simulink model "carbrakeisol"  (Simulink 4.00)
settings: Solver=ode15s  StartTime=0.0  StopTime=Te  RelTol=1e-3
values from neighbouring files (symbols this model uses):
  c1 = 500    [bspbesch.m]    (also in bspofen.m = 921; carbrake.m = 0.857; ffwfback.m = [1 0]; kennwrt.m = 1)
  c2 = 921    [bspbesch.m]    (also in bspofen.m = 465; carbrake.m = 33.822; kennwrt.m = 1; schlupfsoll.m = 33.822)
  c3 = 465    [bspbesch.m]    (also in carbrake.m = 0.347; schlupfsoll.m = 0.347)
  dt = 0.1    [BatchTanks.m]    (also in carbrake.m = 0.01; fensterh.m = 0.005; kennwrt.m = 0.025; ljapst.m = (T(2)-T(1))/20)
  Fb = aSoll*m    [carbrake.m]
  g = 9.81    [autobew.m]    (also in carbrake.m; drifter.m; ffwfback.m; ljapst.m)
  J = m*(ri*ri+ra*ra)/2    (= 24.217)    [carbrake.m]    (also in drehzr.m = 0.0013; fensterh.m = 1.3e-05; motor.m = 0.0013)
  m = 1000    [autobew.m]    (also in Bspreak.m = 10; carbrake.m = 250; drifter.m = 163.8; ffwfback.m = 0.3)
  omega0 = v0/r    (= 34.2090859332)    [carbrake.m]
  r = 0.406    [carbrake.m]    (also in ofenstb.m = [Ad(1,1)+Ad(2,2))
  v = []    [ljapst.m]    (also in omegav2lambda.m = u(1))
  v0 = 50/3.6    (= 13.8888888889)    [carbrake.m]
undefined symbols (not defined in the file or in its folder): omega

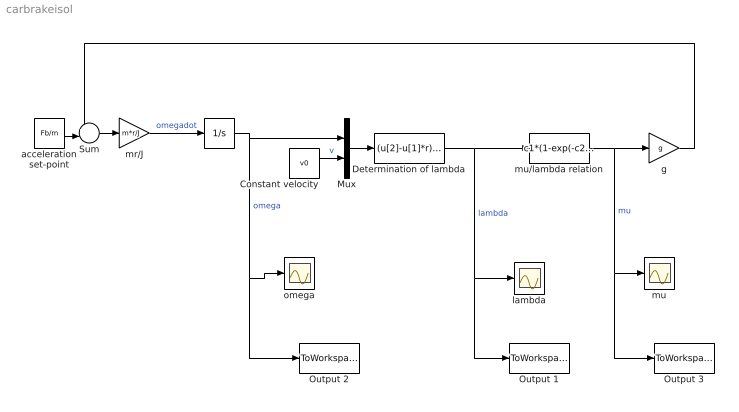
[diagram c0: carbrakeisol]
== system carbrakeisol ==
  " " : Integrator  ExternalReset=none  InitialConditionSource=internal  InitialCondition=omega0  LimitOutput=on  UpperSaturationLimit=inf  LowerSaturationLimit=0  ShowSaturationPort=off  ShowStatePort=off  AbsoluteTolerance=auto
  Constant velocity : Constant  Value=v0
  Determination of lambda : Fcn  Expr=(u[2]-u[1]*r)/u[2]
  Mux : Mux  Inputs=omega,v
  Output 1 : ToWorkspace  VariableName=lambda  SampleTime=dt  SaveFormat=Array
  Output 2 : ToWorkspace  VariableName=omega  SampleTime=dt  SaveFormat=Array
  Output 3 : ToWorkspace  VariableName=mu  SampleTime=dt  SaveFormat=Array
  Sum : Sum  Inputs=+-|  SaturateOnIntegerOverflow=on
  acceleration set-point : Constant  Value=Fb/m
  g : Gain  Gain=g  Multiplication=Element-wise(K.*u)  SaturateOnIntegerOverflow=on
  lambda : Scope
  mr/J : Gain  Gain=m*r/J  Multiplication=Element-wise(K.*u)  SaturateOnIntegerOverflow=on
  mu : Scope
  mu/lambda relation : Fcn  Expr=c1*(1-exp(-c2*u))-c3*u
  omega : Scope
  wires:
  mr/J/1 -> " "/1  "omegadot"
  " "/1 -> Mux/1, omega/1, Output 2/1  "omega"
  Mux/1 -> Determination of lambda/1
  Determination of lambda/1 -> mu/lambda relation/1, lambda/1, Output 1/1  "lambda"
  mu/lambda relation/1 -> g/1, mu/1, Output 3/1  "mu"
  g/1 -> Sum/1
  acceleration set-point/1 -> Sum/2
  Sum/1 -> mr/J/1
  Constant velocity/1 -> Mux/2  "v"
